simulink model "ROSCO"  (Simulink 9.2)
settings: Solver=VariableStepAuto  StartTime=0.0  StopTime=TMax  RelTol=1e-3
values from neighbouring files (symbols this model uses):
  OutList = [OutList    [runFAST.m]    (also in ROSCO2Matlab.m = [])
undefined symbols (not defined in the file or in its folder): cosd, DiscIntNeverNeededParam, F, Parameter, R, rpm2radps, simu, sind, strmatch
libraries: simulink x10
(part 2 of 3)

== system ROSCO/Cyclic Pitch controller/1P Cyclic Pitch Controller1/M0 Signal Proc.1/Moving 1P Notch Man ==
  Input : Inport
  GenSpeedIN : Inport  Port=2
  Gain : Gain  Gain=1/Parameter.Turbine.G * rpm2radps(1)
  Moving 1P Filt Manual : Subsystem
  Slow Low Pass for Param : DiscreteStateSpace  A=Parameter.Control.cIPC.dLPF_slow.a  B=Parameter.Control.cIPC.dLPF_slow.b  C=Parameter.Control.cIPC.dLPF_slow.c  D=Parameter.Control.cIPC.dLPF_slow.d  SampleTime=Parameter.Control.DT
  Output : Outport
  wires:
  GenSpeedIN/1 -> Slow Low Pass for Param/1
  Input/1 -> Moving 1P Filt Manual/1(u)
  Gain/1 -> Moving 1P Filt Manual/2(rot speed (rad/s))
  Slow Low Pass for Param/1 -> Gain/1
  Moving 1P Filt Manual/1(Out1) -> Output/1

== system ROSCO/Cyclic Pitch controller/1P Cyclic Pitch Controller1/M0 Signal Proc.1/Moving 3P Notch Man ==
  Input : Inport
  GenSpeedIN : Inport  Port=2
  Gain : Gain  Gain=1/Parameter.Turbine.G * rpm2radps(1) * 3
  Moving 3P Filt Manual : Subsystem
  Slow Low Pass for Param : DiscreteStateSpace  A=Parameter.Control.cIPC.dLPF_slow.a  B=Parameter.Control.cIPC.dLPF_slow.b  C=Parameter.Control.cIPC.dLPF_slow.c  D=Parameter.Control.cIPC.dLPF_slow.d  SampleTime=Parameter.Control.DT
  Output : Outport
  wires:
  Slow Low Pass for Param/1 -> Gain/1
  Gain/1 -> Moving 3P Filt Manual/2(rot speed (rad/s))
  Input/1 -> Moving 3P Filt Manual/1(u)
  GenSpeedIN/1 -> Slow Low Pass for Param/1
  Moving 3P Filt Manual/1(Out1) -> Output/1

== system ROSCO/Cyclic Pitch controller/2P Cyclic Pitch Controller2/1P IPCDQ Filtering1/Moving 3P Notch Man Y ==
  Input : Inport
  GenSpeedIN : Inport  Port=2
  Gain : Gain  Gain=1/Parameter.Turbine.G * rpm2radps(1) * 3
  Moving 3P Filt Manual : Subsystem
  Slow Low Pass for Param : DiscreteStateSpace  A=Parameter.Control.cIPC.dLPF_slow.a  B=Parameter.Control.cIPC.dLPF_slow.b  C=Parameter.Control.cIPC.dLPF_slow.c  D=Parameter.Control.cIPC.dLPF_slow.d  SampleTime=Parameter.Control.DT
  Output : Outport
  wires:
  Slow Low Pass for Param/1 -> Gain/1
  Gain/1 -> Moving 3P Filt Manual/2(rot speed (rad/s))
  Input/1 -> Moving 3P Filt Manual/1(u)
  GenSpeedIN/1 -> Slow Low Pass for Param/1
  Moving 3P Filt Manual/1(Out1) -> Output/1

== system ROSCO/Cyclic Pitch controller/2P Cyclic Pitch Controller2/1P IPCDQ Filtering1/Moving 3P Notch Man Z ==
  Input : Inport
  GenSpeedIN : Inport  Port=2
  Gain : Gain  Gain=1/Parameter.Turbine.G * rpm2radps(1) * 3
  Moving 3P Filt Manual : Subsystem
  Slow Low Pass for Param : DiscreteStateSpace  A=Parameter.Control.cIPC.dLPF_slow.a  B=Parameter.Control.cIPC.dLPF_slow.b  C=Parameter.Control.cIPC.dLPF_slow.c  D=Parameter.Control.cIPC.dLPF_slow.d  SampleTime=Parameter.Control.DT
  Output : Outport
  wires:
  Moving 3P Filt Manual/1(Out1) -> Output/1
  GenSpeedIN/1 -> Slow Low Pass for Param/1
  Input/1 -> Moving 3P Filt Manual/1(u)
  Gain/1 -> Moving 3P Filt Manual/2(rot speed (rad/s))
  Slow Low Pass for Param/1 -> Gain/1

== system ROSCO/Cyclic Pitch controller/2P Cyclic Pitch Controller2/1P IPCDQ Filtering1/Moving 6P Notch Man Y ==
  Input : Inport
  GenSpeedIN : Inport  Port=2
  Gain : Gain  Gain=1/Parameter.Turbine.G * rpm2radps(1) * 3
  Moving 6P Filt Manual : Subsystem
  Slow Low Pass for Param : DiscreteStateSpace  A=Parameter.Control.cIPC.dLPF_slow.a  B=Parameter.Control.cIPC.dLPF_slow.b  C=Parameter.Control.cIPC.dLPF_slow.c  D=Parameter.Control.cIPC.dLPF_slow.d  SampleTime=Parameter.Control.DT
  Output : Outport
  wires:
  Moving 6P Filt Manual/1(Out1) -> Output/1
  GenSpeedIN/1 -> Slow Low Pass for Param/1
  Input/1 -> Moving 6P Filt Manual/1(u)
  Gain/1 -> Moving 6P Filt Manual/2(rot speed (rad/s))
  Slow Low Pass for Param/1 -> Gain/1

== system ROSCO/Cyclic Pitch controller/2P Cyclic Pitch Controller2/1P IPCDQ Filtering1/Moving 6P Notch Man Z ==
  Input : Inport
  GenSpeedIN : Inport  Port=2
  Gain : Gain  Gain=1/Parameter.Turbine.G * rpm2radps(1) * 3
  Moving 6P Filt Manual : Subsystem
  Slow Low Pass for Param : DiscreteStateSpace  A=Parameter.Control.cIPC.dLPF_slow.a  B=Parameter.Control.cIPC.dLPF_slow.b  C=Parameter.Control.cIPC.dLPF_slow.c  D=Parameter.Control.cIPC.dLPF_slow.d  SampleTime=Parameter.Control.DT
  Output : Outport
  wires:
  Slow Low Pass for Param/1 -> Gain/1
  Gain/1 -> Moving 6P Filt Manual/2(rot speed (rad/s))
  Input/1 -> Moving 6P Filt Manual/1(u)
  GenSpeedIN/1 -> Slow Low Pass for Param/1
  Moving 6P Filt Manual/1(Out1) -> Output/1

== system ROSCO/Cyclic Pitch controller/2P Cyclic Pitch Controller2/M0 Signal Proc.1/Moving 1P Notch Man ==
  Input : Inport
  GenSpeedIN : Inport  Port=2
  Gain : Gain  Gain=1/Parameter.Turbine.G * rpm2radps(1)
  Moving 1P Filt Manual : Subsystem
  Slow Low Pass for Param : DiscreteStateSpace  A=Parameter.Control.cIPC.dLPF_slow.a  B=Parameter.Control.cIPC.dLPF_slow.b  C=Parameter.Control.cIPC.dLPF_slow.c  D=Parameter.Control.cIPC.dLPF_slow.d  SampleTime=Parameter.Control.DT
  Output : Outport
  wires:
  GenSpeedIN/1 -> Slow Low Pass for Param/1
  Input/1 -> Moving 1P Filt Manual/1(u)
  Gain/1 -> Moving 1P Filt Manual/2(rot speed (rad/s))
  Slow Low Pass for Param/1 -> Gain/1
  Moving 1P Filt Manual/1(Out1) -> Output/1

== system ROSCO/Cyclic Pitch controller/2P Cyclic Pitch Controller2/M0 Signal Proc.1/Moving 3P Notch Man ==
  Input : Inport
  GenSpeedIN : Inport  Port=2
  Gain : Gain  Gain=1/Parameter.Turbine.G * rpm2radps(1) * 3
  Moving 3P Filt Manual : Subsystem
  Slow Low Pass for Param : DiscreteStateSpace  A=Parameter.Control.cIPC.dLPF_slow.a  B=Parameter.Control.cIPC.dLPF_slow.b  C=Parameter.Control.cIPC.dLPF_slow.c  D=Parameter.Control.cIPC.dLPF_slow.d  SampleTime=Parameter.Control.DT
  Output : Outport
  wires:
  Slow Low Pass for Param/1 -> Gain/1
  Gain/1 -> Moving 3P Filt Manual/2(rot speed (rad/s))
  Input/1 -> Moving 3P Filt Manual/1(u)
  GenSpeedIN/1 -> Slow Low Pass for Param/1
  Moving 3P Filt Manual/1(Out1) -> Output/1

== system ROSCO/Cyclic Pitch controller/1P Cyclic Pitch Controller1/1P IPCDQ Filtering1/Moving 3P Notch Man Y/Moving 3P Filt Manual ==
  u : Inport
  rot speed (rad/s) : Inport  Port=2
  Den LPV : Subsystem
  Discrete Filter : DiscreteFilter  NumeratorSource=Input port  DenominatorSource=Input port  a0EqualsOne=on
  Num LPV : Subsystem
  Out1 : Outport
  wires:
  u/1 -> Discrete Filter/1
  Num LPV/1(b) -> Discrete Filter/2
  Discrete Filter/1 -> Out1/1
  rot speed (rad/s)/1 -> Den LPV/1(rot speed (rad/s)), Num LPV/1(rot speed (rad/s))
  Den LPV/1(a) -> Discrete Filter/3

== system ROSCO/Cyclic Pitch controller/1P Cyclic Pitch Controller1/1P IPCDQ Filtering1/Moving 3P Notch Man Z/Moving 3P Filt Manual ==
  u : Inport
  rot speed (rad/s) : Inport  Port=2
  Den LPV : Subsystem
  Discrete Filter : DiscreteFilter  NumeratorSource=Input port  DenominatorSource=Input port  a0EqualsOne=on
  Num LPV : Subsystem
  Out1 : Outport
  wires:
  Den LPV/1(a) -> Discrete Filter/3
  rot speed (rad/s)/1 -> Num LPV/1(rot speed (rad/s)), Den LPV/1(rot speed (rad/s))
  Discrete Filter/1 -> Out1/1
  Num LPV/1(b) -> Discrete Filter/2
  u/1 -> Discrete Filter/1

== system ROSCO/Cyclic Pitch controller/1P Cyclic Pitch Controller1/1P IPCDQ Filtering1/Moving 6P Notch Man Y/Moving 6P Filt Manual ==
  u : Inport
  rot speed (rad/s) : Inport  Port=2
  Den LPV : Subsystem
  Discrete Filter : DiscreteFilter  NumeratorSource=Input port  DenominatorSource=Input port  a0EqualsOne=on
  Num LPV : Subsystem
  Out1 : Outport
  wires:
  Den LPV/1(a) -> Discrete Filter/3
  rot speed (rad/s)/1 -> Num LPV/1(rot speed (rad/s)), Den LPV/1(rot speed (rad/s))
  Discrete Filter/1 -> Out1/1
  Num LPV/1(b) -> Discrete Filter/2
  u/1 -> Discrete Filter/1

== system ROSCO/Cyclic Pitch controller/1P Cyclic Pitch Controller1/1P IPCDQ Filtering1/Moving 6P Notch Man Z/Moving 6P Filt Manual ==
  u : Inport
  rot speed (rad/s) : Inport  Port=2
  Den LPV : Subsystem
  Discrete Filter : DiscreteFilter  NumeratorSource=Input port  DenominatorSource=Input port  a0EqualsOne=on
  Num LPV : Subsystem
  Out1 : Outport
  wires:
  u/1 -> Discrete Filter/1
  Num LPV/1(b) -> Discrete Filter/2
  Discrete Filter/1 -> Out1/1
  rot speed (rad/s)/1 -> Den LPV/1(rot speed (rad/s)), Num LPV/1(rot speed (rad/s))
  Den LPV/1(a) -> Discrete Filter/3

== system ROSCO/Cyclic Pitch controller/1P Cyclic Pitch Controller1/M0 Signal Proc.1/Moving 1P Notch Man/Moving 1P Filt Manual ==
  u : Inport
  rot speed (rad/s) : Inport  Port=2
  Den LPV : Subsystem
  Discrete Filter : DiscreteFilter  NumeratorSource=Input port  DenominatorSource=Input port  a0EqualsOne=on
  Num LPV : Subsystem
  Out1 : Outport
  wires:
  Den LPV/1(a) -> Discrete Filter/3
  rot speed (rad/s)/1 -> Num LPV/1(rot speed (rad/s)), Den LPV/1(rot speed (rad/s))
  Discrete Filter/1 -> Out1/1
  Num LPV/1(b) -> Discrete Filter/2
  u/1 -> Discrete Filter/1

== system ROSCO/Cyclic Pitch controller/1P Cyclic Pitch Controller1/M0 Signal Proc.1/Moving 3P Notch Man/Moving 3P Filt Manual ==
  u : Inport
  rot speed (rad/s) : Inport  Port=2
  Den LPV : Subsystem
  Discrete Filter : DiscreteFilter  NumeratorSource=Input port  DenominatorSource=Input port  a0EqualsOne=on
  Num LPV : Subsystem
  Out1 : Outport
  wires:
  u/1 -> Discrete Filter/1
  Num LPV/1(b) -> Discrete Filter/2
  Discrete Filter/1 -> Out1/1
  rot speed (rad/s)/1 -> Den LPV/1(rot speed (rad/s)), Num LPV/1(rot speed (rad/s))
  Den LPV/1(a) -> Discrete Filter/3

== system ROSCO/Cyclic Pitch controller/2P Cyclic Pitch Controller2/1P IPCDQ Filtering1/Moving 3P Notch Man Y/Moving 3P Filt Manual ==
  u : Inport
  rot speed (rad/s) : Inport  Port=2
  Den LPV : Subsystem
  Discrete Filter : DiscreteFilter  NumeratorSource=Input port  DenominatorSource=Input port  a0EqualsOne=on
  Num LPV : Subsystem
  Out1 : Outport
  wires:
  u/1 -> Discrete Filter/1
  Num LPV/1(b) -> Discrete Filter/2
  Discrete Filter/1 -> Out1/1
  rot speed (rad/s)/1 -> Den LPV/1(rot speed (rad/s)), Num LPV/1(rot speed (rad/s))
  Den LPV/1(a) -> Discrete Filter/3

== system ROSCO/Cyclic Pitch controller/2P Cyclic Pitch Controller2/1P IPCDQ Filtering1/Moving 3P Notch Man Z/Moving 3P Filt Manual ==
  u : Inport
  rot speed (rad/s) : Inport  Port=2
  Den LPV : Subsystem
  Discrete Filter : DiscreteFilter  NumeratorSource=Input port  DenominatorSource=Input port  a0EqualsOne=on
  Num LPV : Subsystem
  Out1 : Outport
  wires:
  Den LPV/1(a) -> Discrete Filter/3
  rot speed (rad/s)/1 -> Num LPV/1(rot speed (rad/s)), Den LPV/1(rot speed (rad/s))
  Discrete Filter/1 -> Out1/1
  Num LPV/1(b) -> Discrete Filter/2
  u/1 -> Discrete Filter/1

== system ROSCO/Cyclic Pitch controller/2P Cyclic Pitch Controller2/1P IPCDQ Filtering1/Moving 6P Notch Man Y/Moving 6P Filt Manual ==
  u : Inport
  rot speed (rad/s) : Inport  Port=2
  Den LPV : Subsystem
  Discrete Filter : DiscreteFilter  NumeratorSource=Input port  DenominatorSource=Input port  a0EqualsOne=on
  Num LPV : Subsystem
  Out1 : Outport
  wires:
  Den LPV/1(a) -> Discrete Filter/3
  rot speed (rad/s)/1 -> Num LPV/1(rot speed (rad/s)), Den LPV/1(rot speed (rad/s))
  Discrete Filter/1 -> Out1/1
  Num LPV/1(b) -> Discrete Filter/2
  u/1 -> Discrete Filter/1

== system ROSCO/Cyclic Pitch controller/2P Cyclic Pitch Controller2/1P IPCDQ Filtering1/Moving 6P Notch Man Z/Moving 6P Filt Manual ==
  u : Inport
  rot speed (rad/s) : Inport  Port=2
  Den LPV : Subsystem
  Discrete Filter : DiscreteFilter  NumeratorSource=Input port  DenominatorSource=Input port  a0EqualsOne=on
  Num LPV : Subsystem
  Out1 : Outport
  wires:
  u/1 -> Discrete Filter/1
  Num LPV/1(b) -> Discrete Filter/2
  Discrete Filter/1 -> Out1/1
  rot speed (rad/s)/1 -> Den LPV/1(rot speed (rad/s)), Num LPV/1(rot speed (rad/s))
  Den LPV/1(a) -> Discrete Filter/3

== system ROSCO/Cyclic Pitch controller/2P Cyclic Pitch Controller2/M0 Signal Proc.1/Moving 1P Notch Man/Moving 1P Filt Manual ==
  u : Inport
  rot speed (rad/s) : Inport  Port=2
  Den LPV : Subsystem
  Discrete Filter : DiscreteFilter  NumeratorSource=Input port  DenominatorSource=Input port  a0EqualsOne=on
  Num LPV : Subsystem
  Out1 : Outport
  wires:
  Den LPV/1(a) -> Discrete Filter/3
  rot speed (rad/s)/1 -> Num LPV/1(rot speed (rad/s)), Den LPV/1(rot speed (rad/s))
  Discrete Filter/1 -> Out1/1
  Num LPV/1(b) -> Discrete Filter/2
  u/1 -> Discrete Filter/1

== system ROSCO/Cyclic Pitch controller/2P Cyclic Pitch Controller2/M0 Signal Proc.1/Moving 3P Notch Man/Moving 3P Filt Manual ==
  u : Inport
  rot speed (rad/s) : Inport  Port=2
  Den LPV : Subsystem
  Discrete Filter : DiscreteFilter  NumeratorSource=Input port  DenominatorSource=Input port  a0EqualsOne=on
  Num LPV : Subsystem
  Out1 : Outport
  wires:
  u/1 -> Discrete Filter/1
  Num LPV/1(b) -> Discrete Filter/2
  Discrete Filter/1 -> Out1/1
  rot speed (rad/s)/1 -> Den LPV/1(rot speed (rad/s)), Num LPV/1(rot speed (rad/s))
  Den LPV/1(a) -> Discrete Filter/3

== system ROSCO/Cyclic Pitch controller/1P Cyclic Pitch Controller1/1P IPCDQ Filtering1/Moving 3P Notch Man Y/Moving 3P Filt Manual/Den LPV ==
  rot speed (rad/s) : Inport
  1-D Lookup Table : Lookup_n-D  NumberOfTableDimensions=1  BreakpointsForDimension1=Parameter.Control.cIPC.PSM0_NF_3P.om_3P  BeginIndexSearchUsingPreviousIndexResult=on  Table=Parameter.Control.cIPC.PSM0_NF_3P.a_2  ExtrapMethod=Clip  InternalRulePriority=Speed  RndMeth=Simplest
  1-D Lookup Table1 : Lookup_n-D  NumberOfTableDimensions=1  BreakpointsForDimension1=Parameter.Control.cIPC.PSM0_NF_3P.om_3P  BeginIndexSearchUsingPreviousIndexResult=on  Table=Parameter.Control.cIPC.PSM0_NF_3P.a_1  ExtrapMethod=Clip  InternalRulePriority=Speed  RndMeth=Simplest
  1-D Lookup Table2 : Lookup_n-D  NumberOfTableDimensions=1  BreakpointsForDimension1=Parameter.Control.cIPC.PSM0_NF_3P.om_3P  BeginIndexSearchUsingPreviousIndexResult=on  Table=Parameter.Control.cIPC.PSM0_NF_3P.a_0  ExtrapMethod=Clip  InternalRulePriority=Speed  RndMeth=Simplest
  Mux : Mux  Inputs=3
  a : Outport
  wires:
  1-D Lookup Table/1 -> Mux/1
  1-D Lookup Table1/1 -> Mux/2
  Mux/1 -> a/1
  rot speed (rad/s)/1 -> 1-D Lookup Table2/1, 1-D Lookup Table/1, 1-D Lookup Table1/1
  1-D Lookup Table2/1 -> Mux/3

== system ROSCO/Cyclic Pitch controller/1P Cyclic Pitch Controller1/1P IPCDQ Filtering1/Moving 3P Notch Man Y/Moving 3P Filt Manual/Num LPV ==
  rot speed (rad/s) : Inport
  1-D Lookup Table : Lookup_n-D  NumberOfTableDimensions=1  BreakpointsForDimension1=Parameter.Control.cIPC.PSM0_NF_3P.om_3P  BeginIndexSearchUsingPreviousIndexResult=on  Table=Parameter.Control.cIPC.PSM0_NF_3P.b_2  ExtrapMethod=Clip  InternalRulePriority=Speed  RndMeth=Simplest
  1-D Lookup Table1 : Lookup_n-D  NumberOfTableDimensions=1  BreakpointsForDimension1=Parameter.Control.cIPC.PSM0_NF_3P.om_3P  BeginIndexSearchUsingPreviousIndexResult=on  Table=Parameter.Control.cIPC.PSM0_NF_3P.b_1  ExtrapMethod=Clip  InternalRulePriority=Speed  RndMeth=Simplest
  1-D Lookup Table2 : Lookup_n-D  NumberOfTableDimensions=1  BreakpointsForDimension1=Parameter.Control.cIPC.PSM0_NF_3P.om_3P  BeginIndexSearchUsingPreviousIndexResult=on  Table=Parameter.Control.cIPC.PSM0_NF_3P.b_0  ExtrapMethod=Clip  InternalRulePriority=Speed  RndMeth=Simplest
  Mux : Mux  Inputs=3
  b : Outport
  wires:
  1-D Lookup Table2/1 -> Mux/3
  rot speed (rad/s)/1 -> 1-D Lookup Table1/1, 1-D Lookup Table/1, 1-D Lookup Table2/1
  Mux/1 -> b/1
  1-D Lookup Table1/1 -> Mux/2
  1-D Lookup Table/1 -> Mux/1

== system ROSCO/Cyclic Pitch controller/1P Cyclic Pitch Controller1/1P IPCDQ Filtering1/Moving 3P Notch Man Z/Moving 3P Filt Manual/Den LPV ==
  rot speed (rad/s) : Inport
  1-D Lookup Table : Lookup_n-D  NumberOfTableDimensions=1  BreakpointsForDimension1=Parameter.Control.cIPC.PSM0_NF_3P.om_3P  BeginIndexSearchUsingPreviousIndexResult=on  Table=Parameter.Control.cIPC.PSM0_NF_3P.a_2  ExtrapMethod=Clip  InternalRulePriority=Speed  RndMeth=Simplest
  1-D Lookup Table1 : Lookup_n-D  NumberOfTableDimensions=1  BreakpointsForDimension1=Parameter.Control.cIPC.PSM0_NF_3P.om_3P  BeginIndexSearchUsingPreviousIndexResult=on  Table=Parameter.Control.cIPC.PSM0_NF_3P.a_1  ExtrapMethod=Clip  InternalRulePriority=Speed  RndMeth=Simplest
  1-D Lookup Table2 : Lookup_n-D  NumberOfTableDimensions=1  BreakpointsForDimension1=Parameter.Control.cIPC.PSM0_NF_3P.om_3P  BeginIndexSearchUsingPreviousIndexResult=on  Table=Parameter.Control.cIPC.PSM0_NF_3P.a_0  ExtrapMethod=Clip  InternalRulePriority=Speed  RndMeth=Simplest
  Mux : Mux  Inputs=3
  a : Outport
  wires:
  1-D Lookup Table2/1 -> Mux/3
  rot speed (rad/s)/1 -> 1-D Lookup Table1/1, 1-D Lookup Table/1, 1-D Lookup Table2/1
  Mux/1 -> a/1
  1-D Lookup Table1/1 -> Mux/2
  1-D Lookup Table/1 -> Mux/1

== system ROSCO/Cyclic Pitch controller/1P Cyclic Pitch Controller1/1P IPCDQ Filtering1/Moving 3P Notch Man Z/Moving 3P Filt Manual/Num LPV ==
  rot speed (rad/s) : Inport
  1-D Lookup Table : Lookup_n-D  NumberOfTableDimensions=1  BreakpointsForDimension1=Parameter.Control.cIPC.PSM0_NF_3P.om_3P  BeginIndexSearchUsingPreviousIndexResult=on  Table=Parameter.Control.cIPC.PSM0_NF_3P.b_2  ExtrapMethod=Clip  InternalRulePriority=Speed  RndMeth=Simplest
  1-D Lookup Table1 : Lookup_n-D  NumberOfTableDimensions=1  BreakpointsForDimension1=Parameter.Control.cIPC.PSM0_NF_3P.om_3P  BeginIndexSearchUsingPreviousIndexResult=on  Table=Parameter.Control.cIPC.PSM0_NF_3P.b_1  ExtrapMethod=Clip  InternalRulePriority=Speed  RndMeth=Simplest
  1-D Lookup Table2 : Lookup_n-D  NumberOfTableDimensions=1  BreakpointsForDimension1=Parameter.Control.cIPC.PSM0_NF_3P.om_3P  BeginIndexSearchUsingPreviousIndexResult=on  Table=Parameter.Control.cIPC.PSM0_NF_3P.b_0  ExtrapMethod=Clip  InternalRulePriority=Speed  RndMeth=Simplest
  Mux : Mux  Inputs=3
  b : Outport
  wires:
  1-D Lookup Table/1 -> Mux/1
  1-D Lookup Table1/1 -> Mux/2
  Mux/1 -> b/1
  rot speed (rad/s)/1 -> 1-D Lookup Table2/1, 1-D Lookup Table/1, 1-D Lookup Table1/1
  1-D Lookup Table2/1 -> Mux/3

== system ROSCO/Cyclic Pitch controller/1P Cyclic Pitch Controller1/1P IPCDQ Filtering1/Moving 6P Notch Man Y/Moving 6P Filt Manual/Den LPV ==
  rot speed (rad/s) : Inport
  1-D Lookup Table : Lookup_n-D  NumberOfTableDimensions=1  BreakpointsForDimension1=Parameter.Control.cIPC.PSM0_NF_6P.om_6P  BeginIndexSearchUsingPreviousIndexResult=on  Table=Parameter.Control.cIPC.PSM0_NF_6P.a_2  ExtrapMethod=Clip  InternalRulePriority=Speed  RndMeth=Simplest
  1-D Lookup Table1 : Lookup_n-D  NumberOfTableDimensions=1  BreakpointsForDimension1=Parameter.Control.cIPC.PSM0_NF_6P.om_6P  BeginIndexSearchUsingPreviousIndexResult=on  Table=Parameter.Control.cIPC.PSM0_NF_6P.a_1  ExtrapMethod=Clip  InternalRulePriority=Speed  RndMeth=Simplest
  1-D Lookup Table2 : Lookup_n-D  NumberOfTableDimensions=1  BreakpointsForDimension1=Parameter.Control.cIPC.PSM0_NF_6P.om_6P  BeginIndexSearchUsingPreviousIndexResult=on  Table=Parameter.Control.cIPC.PSM0_NF_6P.a_0  ExtrapMethod=Clip  InternalRulePriority=Speed  RndMeth=Simplest
  Mux : Mux  Inputs=3
  a : Outport
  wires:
  1-D Lookup Table2/1 -> Mux/3
  rot speed (rad/s)/1 -> 1-D Lookup Table1/1, 1-D Lookup Table/1, 1-D Lookup Table2/1
  Mux/1 -> a/1
  1-D Lookup Table1/1 -> Mux/2
  1-D Lookup Table/1 -> Mux/1

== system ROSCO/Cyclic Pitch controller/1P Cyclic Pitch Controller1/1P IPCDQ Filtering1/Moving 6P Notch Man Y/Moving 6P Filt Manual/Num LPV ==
  rot speed (rad/s) : Inport
  1-D Lookup Table : Lookup_n-D  NumberOfTableDimensions=1  BreakpointsForDimension1=Parameter.Control.cIPC.PSM0_NF_6P.om_6P  BeginIndexSearchUsingPreviousIndexResult=on  Table=Parameter.Control.cIPC.PSM0_NF_6P.b_2  ExtrapMethod=Clip  InternalRulePriority=Speed  RndMeth=Simplest
  1-D Lookup Table1 : Lookup_n-D  NumberOfTableDimensions=1  BreakpointsForDimension1=Parameter.Control.cIPC.PSM0_NF_6P.om_6P  BeginIndexSearchUsingPreviousIndexResult=on  Table=Parameter.Control.cIPC.PSM0_NF_6P.b_1  ExtrapMethod=Clip  InternalRulePriority=Speed  RndMeth=Simplest
  1-D Lookup Table2 : Lookup_n-D  NumberOfTableDimensions=1  BreakpointsForDimension1=Parameter.Control.cIPC.PSM0_NF_6P.om_6P  BeginIndexSearchUsingPreviousIndexResult=on  Table=Parameter.Control.cIPC.PSM0_NF_6P.b_0  ExtrapMethod=Clip  InternalRulePriority=Speed  RndMeth=Simplest
  Mux : Mux  Inputs=3
  b : Outport
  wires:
  1-D Lookup Table/1 -> Mux/1
  1-D Lookup Table1/1 -> Mux/2
  Mux/1 -> b/1
  rot speed (rad/s)/1 -> 1-D Lookup Table2/1, 1-D Lookup Table1/1, 1-D Lookup Table/1
  1-D Lookup Table2/1 -> Mux/3

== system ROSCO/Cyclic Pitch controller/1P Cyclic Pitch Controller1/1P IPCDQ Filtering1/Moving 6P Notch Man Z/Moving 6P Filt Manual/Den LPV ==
  rot speed (rad/s) : Inport
  1-D Lookup Table : Lookup_n-D  NumberOfTableDimensions=1  BreakpointsForDimension1=Parameter.Control.cIPC.PSM0_NF_6P.om_6P  BeginIndexSearchUsingPreviousIndexResult=on  Table=Parameter.Control.cIPC.PSM0_NF_6P.a_2  ExtrapMethod=Clip  InternalRulePriority=Speed  RndMeth=Simplest
  1-D Lookup Table1 : Lookup_n-D  NumberOfTableDimensions=1  BreakpointsForDimension1=Parameter.Control.cIPC.PSM0_NF_6P.om_6P  BeginIndexSearchUsingPreviousIndexResult=on  Table=Parameter.Control.cIPC.PSM0_NF_6P.a_1  ExtrapMethod=Clip  InternalRulePriority=Speed  RndMeth=Simplest
  1-D Lookup Table2 : Lookup_n-D  NumberOfTableDimensions=1  BreakpointsForDimension1=Parameter.Control.cIPC.PSM0_NF_6P.om_6P  BeginIndexSearchUsingPreviousIndexResult=on  Table=Parameter.Control.cIPC.PSM0_NF_6P.a_0  ExtrapMethod=Clip  InternalRulePriority=Speed  RndMeth=Simplest
  Mux : Mux  Inputs=3
  a : Outport
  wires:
  1-D Lookup Table/1 -> Mux/1
  1-D Lookup Table1/1 -> Mux/2
  Mux/1 -> a/1
  rot speed (rad/s)/1 -> 1-D Lookup Table2/1, 1-D Lookup Table/1, 1-D Lookup Table1/1
  1-D Lookup Table2/1 -> Mux/3

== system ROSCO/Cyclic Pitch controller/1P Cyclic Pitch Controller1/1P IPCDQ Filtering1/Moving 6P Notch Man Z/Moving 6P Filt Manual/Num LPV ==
  rot speed (rad/s) : Inport
  1-D Lookup Table : Lookup_n-D  NumberOfTableDimensions=1  BreakpointsForDimension1=Parameter.Control.cIPC.PSM0_NF_6P.om_6P  BeginIndexSearchUsingPreviousIndexResult=on  Table=Parameter.Control.cIPC.PSM0_NF_6P.b_2  ExtrapMethod=Clip  InternalRulePriority=Speed  RndMeth=Simplest
  1-D Lookup Table1 : Lookup_n-D  NumberOfTableDimensions=1  BreakpointsForDimension1=Parameter.Control.cIPC.PSM0_NF_6P.om_6P  BeginIndexSearchUsingPreviousIndexResult=on  Table=Parameter.Control.cIPC.PSM0_NF_6P.b_1  ExtrapMethod=Clip  InternalRulePriority=Speed  RndMeth=Simplest
  1-D Lookup Table2 : Lookup_n-D  NumberOfTableDimensions=1  BreakpointsForDimension1=Parameter.Control.cIPC.PSM0_NF_6P.om_6P  BeginIndexSearchUsingPreviousIndexResult=on  Table=Parameter.Control.cIPC.PSM0_NF_6P.b_0  ExtrapMethod=Clip  InternalRulePriority=Speed  RndMeth=Simplest
  Mux : Mux  Inputs=3
  b : Outport
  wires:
  1-D Lookup Table2/1 -> Mux/3
  rot speed (rad/s)/1 -> 1-D Lookup Table1/1, 1-D Lookup Table/1, 1-D Lookup Table2/1
  Mux/1 -> b/1
  1-D Lookup Table1/1 -> Mux/2
  1-D Lookup Table/1 -> Mux/1

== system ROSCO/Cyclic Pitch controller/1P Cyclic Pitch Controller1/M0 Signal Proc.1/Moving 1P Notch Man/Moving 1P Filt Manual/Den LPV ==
  rot speed (rad/s) : Inport
  1-D Lookup Table : Lookup_n-D  NumberOfTableDimensions=1  BreakpointsForDimension1=Parameter.Control.cIPC.PSM0_NF_1P.om_1P  BeginIndexSearchUsingPreviousIndexResult=on  Table=Parameter.Control.cIPC.PSM0_NF_1P.a_2  ExtrapMethod=Clip  InternalRulePriority=Speed  RndMeth=Simplest
  1-D Lookup Table1 : Lookup_n-D  NumberOfTableDimensions=1  BreakpointsForDimension1=Parameter.Control.cIPC.PSM0_NF_1P.om_1P  BeginIndexSearchUsingPreviousIndexResult=on  Table=Parameter.Control.cIPC.PSM0_NF_1P.a_1  ExtrapMethod=Clip  InternalRulePriority=Speed  RndMeth=Simplest
  1-D Lookup Table2 : Lookup_n-D  NumberOfTableDimensions=1  BreakpointsForDimension1=Parameter.Control.cIPC.PSM0_NF_1P.om_1P  BeginIndexSearchUsingPreviousIndexResult=on  Table=Parameter.Control.cIPC.PSM0_NF_1P.a_0  ExtrapMethod=Clip  InternalRulePriority=Speed  RndMeth=Simplest
  Mux : Mux  Inputs=3
  a : Outport
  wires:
  1-D Lookup Table2/1 -> Mux/3
  rot speed (rad/s)/1 -> 1-D Lookup Table1/1, 1-D Lookup Table/1, 1-D Lookup Table2/1
  Mux/1 -> a/1
  1-D Lookup Table1/1 -> Mux/2
  1-D Lookup Table/1 -> Mux/1

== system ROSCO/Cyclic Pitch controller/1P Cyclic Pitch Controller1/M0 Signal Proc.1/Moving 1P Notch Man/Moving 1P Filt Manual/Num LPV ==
  rot speed (rad/s) : Inport
  1-D Lookup Table : Lookup_n-D  NumberOfTableDimensions=1  BreakpointsForDimension1=Parameter.Control.cIPC.PSM0_NF_1P.om_1P  BeginIndexSearchUsingPreviousIndexResult=on  Table=Parameter.Control.cIPC.PSM0_NF_1P.b_2  ExtrapMethod=Clip  InternalRulePriority=Speed  RndMeth=Simplest
  1-D Lookup Table1 : Lookup_n-D  NumberOfTableDimensions=1  BreakpointsForDimension1=Parameter.Control.cIPC.PSM0_NF_1P.om_1P  BeginIndexSearchUsingPreviousIndexResult=on  Table=Parameter.Control.cIPC.PSM0_NF_1P.b_1  ExtrapMethod=Clip  InternalRulePriority=Speed  RndMeth=Simplest
  1-D Lookup Table2 : Lookup_n-D  NumberOfTableDimensions=1  BreakpointsForDimension1=Parameter.Control.cIPC.PSM0_NF_1P.om_1P  BeginIndexSearchUsingPreviousIndexResult=on  Table=Parameter.Control.cIPC.PSM0_NF_1P.b_0  ExtrapMethod=Clip  InternalRulePriority=Speed  RndMeth=Simplest
  Mux : Mux  Inputs=3
  b : Outport
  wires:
  1-D Lookup Table/1 -> Mux/1
  1-D Lookup Table1/1 -> Mux/2
  Mux/1 -> b/1
  rot speed (rad/s)/1 -> 1-D Lookup Table2/1, 1-D Lookup Table/1, 1-D Lookup Table1/1
  1-D Lookup Table2/1 -> Mux/3

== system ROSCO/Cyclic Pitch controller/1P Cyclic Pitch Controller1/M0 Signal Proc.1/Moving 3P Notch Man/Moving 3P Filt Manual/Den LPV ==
  rot speed (rad/s) : Inport
  1-D Lookup Table : Lookup_n-D  NumberOfTableDimensions=1  BreakpointsForDimension1=Parameter.Control.cIPC.PSM0_NF_3P.om_3P  BeginIndexSearchUsingPreviousIndexResult=on  Table=Parameter.Control.cIPC.PSM0_NF_3P.a_2  ExtrapMethod=Clip  InternalRulePriority=Speed  RndMeth=Simplest
  1-D Lookup Table1 : Lookup_n-D  NumberOfTableDimensions=1  BreakpointsForDimension1=Parameter.Control.cIPC.PSM0_NF_3P.om_3P  BeginIndexSearchUsingPreviousIndexResult=on  Table=Parameter.Control.cIPC.PSM0_NF_3P.a_1  ExtrapMethod=Clip  InternalRulePriority=Speed  RndMeth=Simplest
  1-D Lookup Table2 : Lookup_n-D  NumberOfTableDimensions=1  BreakpointsForDimension1=Parameter.Control.cIPC.PSM0_NF_3P.om_3P  BeginIndexSearchUsingPreviousIndexResult=on  Table=Parameter.Control.cIPC.PSM0_NF_3P.a_0  ExtrapMethod=Clip  InternalRulePriority=Speed  RndMeth=Simplest
  Mux : Mux  Inputs=3
  a : Outport
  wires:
  1-D Lookup Table/1 -> Mux/1
  1-D Lookup Table1/1 -> Mux/2
  Mux/1 -> a/1
  rot speed (rad/s)/1 -> 1-D Lookup Table2/1, 1-D Lookup Table/1, 1-D Lookup Table1/1
  1-D Lookup Table2/1 -> Mux/3

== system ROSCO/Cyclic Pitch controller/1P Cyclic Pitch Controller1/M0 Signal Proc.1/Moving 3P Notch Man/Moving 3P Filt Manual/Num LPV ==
  rot speed (rad/s) : Inport
  1-D Lookup Table : Lookup_n-D  NumberOfTableDimensions=1  BreakpointsForDimension1=Parameter.Control.cIPC.PSM0_NF_3P.om_3P  BeginIndexSearchUsingPreviousIndexResult=on  Table=Parameter.Control.cIPC.PSM0_NF_3P.b_2  ExtrapMethod=Clip  InternalRulePriority=Speed  RndMeth=Simplest
  1-D Lookup Table1 : Lookup_n-D  NumberOfTableDimensions=1  BreakpointsForDimension1=Parameter.Control.cIPC.PSM0_NF_3P.om_3P  BeginIndexSearchUsingPreviousIndexResult=on  Table=Parameter.Control.cIPC.PSM0_NF_3P.b_1  ExtrapMethod=Clip  InternalRulePriority=Speed  RndMeth=Simplest
  1-D Lookup Table2 : Lookup_n-D  NumberOfTableDimensions=1  BreakpointsForDimension1=Parameter.Control.cIPC.PSM0_NF_3P.om_3P  BeginIndexSearchUsingPreviousIndexResult=on  Table=Parameter.Control.cIPC.PSM0_NF_3P.b_0  ExtrapMethod=Clip  InternalRulePriority=Speed  RndMeth=Simplest
  Mux : Mux  Inputs=3
  b : Outport
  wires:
  1-D Lookup Table2/1 -> Mux/3
  rot speed (rad/s)/1 -> 1-D Lookup Table1/1, 1-D Lookup Table/1, 1-D Lookup Table2/1
  Mux/1 -> b/1
  1-D Lookup Table1/1 -> Mux/2
  1-D Lookup Table/1 -> Mux/1

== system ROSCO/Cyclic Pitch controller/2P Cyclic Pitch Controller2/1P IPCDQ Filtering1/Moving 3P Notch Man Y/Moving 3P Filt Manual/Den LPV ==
  rot speed (rad/s) : Inport
  1-D Lookup Table : Lookup_n-D  NumberOfTableDimensions=1  BreakpointsForDimension1=Parameter.Control.cIPC.PSM0_NF_3P.om_3P  BeginIndexSearchUsingPreviousIndexResult=on  Table=Parameter.Control.cIPC.PSM0_NF_3P.a_2  ExtrapMethod=Clip  InternalRulePriority=Speed  RndMeth=Simplest
  1-D Lookup Table1 : Lookup_n-D  NumberOfTableDimensions=1  BreakpointsForDimension1=Parameter.Control.cIPC.PSM0_NF_3P.om_3P  BeginIndexSearchUsingPreviousIndexResult=on  Table=Parameter.Control.cIPC.PSM0_NF_3P.a_1  ExtrapMethod=Clip  InternalRulePriority=Speed  RndMeth=Simplest
  1-D Lookup Table2 : Lookup_n-D  NumberOfTableDimensions=1  BreakpointsForDimension1=Parameter.Control.cIPC.PSM0_NF_3P.om_3P  BeginIndexSearchUsingPreviousIndexResult=on  Table=Parameter.Control.cIPC.PSM0_NF_3P.a_0  ExtrapMethod=Clip  InternalRulePriority=Speed  RndMeth=Simplest
  Mux : Mux  Inputs=3
  a : Outport
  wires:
  1-D Lookup Table/1 -> Mux/1
  1-D Lookup Table1/1 -> Mux/2
  Mux/1 -> a/1
  rot speed (rad/s)/1 -> 1-D Lookup Table2/1, 1-D Lookup Table/1, 1-D Lookup Table1/1
  1-D Lookup Table2/1 -> Mux/3

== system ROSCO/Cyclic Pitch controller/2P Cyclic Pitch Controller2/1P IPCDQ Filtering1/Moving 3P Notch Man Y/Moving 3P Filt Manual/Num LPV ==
  rot speed (rad/s) : Inport
  1-D Lookup Table : Lookup_n-D  NumberOfTableDimensions=1  BreakpointsForDimension1=Parameter.Control.cIPC.PSM0_NF_3P.om_3P  BeginIndexSearchUsingPreviousIndexResult=on  Table=Parameter.Control.cIPC.PSM0_NF_3P.b_2  ExtrapMethod=Clip  InternalRulePriority=Speed  RndMeth=Simplest
  1-D Lookup Table1 : Lookup_n-D  NumberOfTableDimensions=1  BreakpointsForDimension1=Parameter.Control.cIPC.PSM0_NF_3P.om_3P  BeginIndexSearchUsingPreviousIndexResult=on  Table=Parameter.Control.cIPC.PSM0_NF_3P.b_1  ExtrapMethod=Clip  InternalRulePriority=Speed  RndMeth=Simplest
  1-D Lookup Table2 : Lookup_n-D  NumberOfTableDimensions=1  BreakpointsForDimension1=Parameter.Control.cIPC.PSM0_NF_3P.om_3P  BeginIndexSearchUsingPreviousIndexResult=on  Table=Parameter.Control.cIPC.PSM0_NF_3P.b_0  ExtrapMethod=Clip  InternalRulePriority=Speed  RndMeth=Simplest
  Mux : Mux  Inputs=3
  b : Outport
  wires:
  1-D Lookup Table2/1 -> Mux/3
  rot speed (rad/s)/1 -> 1-D Lookup Table1/1, 1-D Lookup Table/1, 1-D Lookup Table2/1
  Mux/1 -> b/1
  1-D Lookup Table1/1 -> Mux/2
  1-D Lookup Table/1 -> Mux/1

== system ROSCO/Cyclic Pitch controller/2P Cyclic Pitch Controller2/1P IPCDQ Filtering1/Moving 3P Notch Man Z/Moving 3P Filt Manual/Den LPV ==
  rot speed (rad/s) : Inport
  1-D Lookup Table : Lookup_n-D  NumberOfTableDimensions=1  BreakpointsForDimension1=Parameter.Control.cIPC.PSM0_NF_3P.om_3P  BeginIndexSearchUsingPreviousIndexResult=on  Table=Parameter.Control.cIPC.PSM0_NF_3P.a_2  ExtrapMethod=Clip  InternalRulePriority=Speed  RndMeth=Simplest
  1-D Lookup Table1 : Lookup_n-D  NumberOfTableDimensions=1  BreakpointsForDimension1=Parameter.Control.cIPC.PSM0_NF_3P.om_3P  BeginIndexSearchUsingPreviousIndexResult=on  Table=Parameter.Control.cIPC.PSM0_NF_3P.a_1  ExtrapMethod=Clip  InternalRulePriority=Speed  RndMeth=Simplest
  1-D Lookup Table2 : Lookup_n-D  NumberOfTableDimensions=1  BreakpointsForDimension1=Parameter.Control.cIPC.PSM0_NF_3P.om_3P  BeginIndexSearchUsingPreviousIndexResult=on  Table=Parameter.Control.cIPC.PSM0_NF_3P.a_0  ExtrapMethod=Clip  InternalRulePriority=Speed  RndMeth=Simplest
  Mux : Mux  Inputs=3
  a : Outport
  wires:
  1-D Lookup Table2/1 -> Mux/3
  rot speed (rad/s)/1 -> 1-D Lookup Table1/1, 1-D Lookup Table/1, 1-D Lookup Table2/1
  Mux/1 -> a/1
  1-D Lookup Table1/1 -> Mux/2
  1-D Lookup Table/1 -> Mux/1

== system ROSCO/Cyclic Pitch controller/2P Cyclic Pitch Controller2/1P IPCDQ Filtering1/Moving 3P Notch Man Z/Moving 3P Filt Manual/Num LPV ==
  rot speed (rad/s) : Inport
  1-D Lookup Table : Lookup_n-D  NumberOfTableDimensions=1  BreakpointsForDimension1=Parameter.Control.cIPC.PSM0_NF_3P.om_3P  BeginIndexSearchUsingPreviousIndexResult=on  Table=Parameter.Control.cIPC.PSM0_NF_3P.b_2  ExtrapMethod=Clip  InternalRulePriority=Speed  RndMeth=Simplest
  1-D Lookup Table1 : Lookup_n-D  NumberOfTableDimensions=1  BreakpointsForDimension1=Parameter.Control.cIPC.PSM0_NF_3P.om_3P  BeginIndexSearchUsingPreviousIndexResult=on  Table=Parameter.Control.cIPC.PSM0_NF_3P.b_1  ExtrapMethod=Clip  InternalRulePriority=Speed  RndMeth=Simplest
  1-D Lookup Table2 : Lookup_n-D  NumberOfTableDimensions=1  BreakpointsForDimension1=Parameter.Control.cIPC.PSM0_NF_3P.om_3P  BeginIndexSearchUsingPreviousIndexResult=on  Table=Parameter.Control.cIPC.PSM0_NF_3P.b_0  ExtrapMethod=Clip  InternalRulePriority=Speed  RndMeth=Simplest
  Mux : Mux  Inputs=3
  b : Outport
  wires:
  1-D Lookup Table/1 -> Mux/1
  1-D Lookup Table1/1 -> Mux/2
  Mux/1 -> b/1
  rot speed (rad/s)/1 -> 1-D Lookup Table2/1, 1-D Lookup Table/1, 1-D Lookup Table1/1
  1-D Lookup Table2/1 -> Mux/3

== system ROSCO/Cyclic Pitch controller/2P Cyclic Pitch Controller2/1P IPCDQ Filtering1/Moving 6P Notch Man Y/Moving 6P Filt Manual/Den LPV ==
  rot speed (rad/s) : Inport
  1-D Lookup Table : Lookup_n-D  NumberOfTableDimensions=1  BreakpointsForDimension1=Parameter.Control.cIPC.PSM0_NF_6P.om_6P  BeginIndexSearchUsingPreviousIndexResult=on  Table=Parameter.Control.cIPC.PSM0_NF_6P.a_2  ExtrapMethod=Clip  InternalRulePriority=Speed  RndMeth=Simplest
  1-D Lookup Table1 : Lookup_n-D  NumberOfTableDimensions=1  BreakpointsForDimension1=Parameter.Control.cIPC.PSM0_NF_6P.om_6P  BeginIndexSearchUsingPreviousIndexResult=on  Table=Parameter.Control.cIPC.PSM0_NF_6P.a_1  ExtrapMethod=Clip  InternalRulePriority=Speed  RndMeth=Simplest
  1-D Lookup Table2 : Lookup_n-D  NumberOfTableDimensions=1  BreakpointsForDimension1=Parameter.Control.cIPC.PSM0_NF_6P.om_6P  BeginIndexSearchUsingPreviousIndexResult=on  Table=Parameter.Control.cIPC.PSM0_NF_6P.a_0  ExtrapMethod=Clip  InternalRulePriority=Speed  RndMeth=Simplest
  Mux : Mux  Inputs=3
  a : Outport
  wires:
  1-D Lookup Table2/1 -> Mux/3
  rot speed (rad/s)/1 -> 1-D Lookup Table1/1, 1-D Lookup Table/1, 1-D Lookup Table2/1
  Mux/1 -> a/1
  1-D Lookup Table1/1 -> Mux/2
  1-D Lookup Table/1 -> Mux/1

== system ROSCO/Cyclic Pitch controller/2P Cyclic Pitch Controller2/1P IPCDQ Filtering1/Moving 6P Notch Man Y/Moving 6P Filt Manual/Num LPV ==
  rot speed (rad/s) : Inport
  1-D Lookup Table : Lookup_n-D  NumberOfTableDimensions=1  BreakpointsForDimension1=Parameter.Control.cIPC.PSM0_NF_6P.om_6P  BeginIndexSearchUsingPreviousIndexResult=on  Table=Parameter.Control.cIPC.PSM0_NF_6P.b_2  ExtrapMethod=Clip  InternalRulePriority=Speed  RndMeth=Simplest
  1-D Lookup Table1 : Lookup_n-D  NumberOfTableDimensions=1  BreakpointsForDimension1=Parameter.Control.cIPC.PSM0_NF_6P.om_6P  BeginIndexSearchUsingPreviousIndexResult=on  Table=Parameter.Control.cIPC.PSM0_NF_6P.b_1  ExtrapMethod=Clip  InternalRulePriority=Speed  RndMeth=Simplest
  1-D Lookup Table2 : Lookup_n-D  NumberOfTableDimensions=1  BreakpointsForDimension1=Parameter.Control.cIPC.PSM0_NF_6P.om_6P  BeginIndexSearchUsingPreviousIndexResult=on  Table=Parameter.Control.cIPC.PSM0_NF_6P.b_0  ExtrapMethod=Clip  InternalRulePriority=Speed  RndMeth=Simplest
  Mux : Mux  Inputs=3
  b : Outport
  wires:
  1-D Lookup Table/1 -> Mux/1
  1-D Lookup Table1/1 -> Mux/2
  Mux/1 -> b/1
  rot speed (rad/s)/1 -> 1-D Lookup Table2/1, 1-D Lookup Table1/1, 1-D Lookup Table/1
  1-D Lookup Table2/1 -> Mux/3

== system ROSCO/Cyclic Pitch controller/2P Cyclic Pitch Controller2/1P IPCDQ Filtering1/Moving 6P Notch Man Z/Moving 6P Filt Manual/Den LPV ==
  rot speed (rad/s) : Inport
  1-D Lookup Table : Lookup_n-D  NumberOfTableDimensions=1  BreakpointsForDimension1=Parameter.Control.cIPC.PSM0_NF_6P.om_6P  BeginIndexSearchUsingPreviousIndexResult=on  Table=Parameter.Control.cIPC.PSM0_NF_6P.a_2  ExtrapMethod=Clip  InternalRulePriority=Speed  RndMeth=Simplest
  1-D Lookup Table1 : Lookup_n-D  NumberOfTableDimensions=1  BreakpointsForDimension1=Parameter.Control.cIPC.PSM0_NF_6P.om_6P  BeginIndexSearchUsingPreviousIndexResult=on  Table=Parameter.Control.cIPC.PSM0_NF_6P.a_1  ExtrapMethod=Clip  InternalRulePriority=Speed  RndMeth=Simplest
  1-D Lookup Table2 : Lookup_n-D  NumberOfTableDimensions=1  BreakpointsForDimension1=Parameter.Control.cIPC.PSM0_NF_6P.om_6P  BeginIndexSearchUsingPreviousIndexResult=on  Table=Parameter.Control.cIPC.PSM0_NF_6P.a_0  ExtrapMethod=Clip  InternalRulePriority=Speed  RndMeth=Simplest
  Mux : Mux  Inputs=3
  a : Outport
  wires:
  1-D Lookup Table/1 -> Mux/1
  1-D Lookup Table1/1 -> Mux/2
  Mux/1 -> a/1
  rot speed (rad/s)/1 -> 1-D Lookup Table2/1, 1-D Lookup Table/1, 1-D Lookup Table1/1
  1-D Lookup Table2/1 -> Mux/3

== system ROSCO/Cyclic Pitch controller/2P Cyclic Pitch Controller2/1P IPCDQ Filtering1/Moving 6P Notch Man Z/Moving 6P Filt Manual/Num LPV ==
  rot speed (rad/s) : Inport
  1-D Lookup Table : Lookup_n-D  NumberOfTableDimensions=1  BreakpointsForDimension1=Parameter.Control.cIPC.PSM0_NF_6P.om_6P  BeginIndexSearchUsingPreviousIndexResult=on  Table=Parameter.Control.cIPC.PSM0_NF_6P.b_2  ExtrapMethod=Clip  InternalRulePriority=Speed  RndMeth=Simplest
  1-D Lookup Table1 : Lookup_n-D  NumberOfTableDimensions=1  BreakpointsForDimension1=Parameter.Control.cIPC.PSM0_NF_6P.om_6P  BeginIndexSearchUsingPreviousIndexResult=on  Table=Parameter.Control.cIPC.PSM0_NF_6P.b_1  ExtrapMethod=Clip  InternalRulePriority=Speed  RndMeth=Simplest
  1-D Lookup Table2 : Lookup_n-D  NumberOfTableDimensions=1  BreakpointsForDimension1=Parameter.Control.cIPC.PSM0_NF_6P.om_6P  BeginIndexSearchUsingPreviousIndexResult=on  Table=Parameter.Control.cIPC.PSM0_NF_6P.b_0  ExtrapMethod=Clip  InternalRulePriority=Speed  RndMeth=Simplest
  Mux : Mux  Inputs=3
  b : Outport
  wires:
  1-D Lookup Table2/1 -> Mux/3
  rot speed (rad/s)/1 -> 1-D Lookup Table1/1, 1-D Lookup Table/1, 1-D Lookup Table2/1
  Mux/1 -> b/1
  1-D Lookup Table1/1 -> Mux/2
  1-D Lookup Table/1 -> Mux/1

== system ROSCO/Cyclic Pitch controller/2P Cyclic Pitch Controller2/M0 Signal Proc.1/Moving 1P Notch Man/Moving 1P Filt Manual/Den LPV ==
  rot speed (rad/s) : Inport
  1-D Lookup Table : Lookup_n-D  NumberOfTableDimensions=1  BreakpointsForDimension1=Parameter.Control.cIPC.PSM0_NF_1P.om_1P  BeginIndexSearchUsingPreviousIndexResult=on  Table=Parameter.Control.cIPC.PSM0_NF_1P.a_2  ExtrapMethod=Clip  InternalRulePriority=Speed  RndMeth=Simplest
  1-D Lookup Table1 : Lookup_n-D  NumberOfTableDimensions=1  BreakpointsForDimension1=Parameter.Control.cIPC.PSM0_NF_1P.om_1P  BeginIndexSearchUsingPreviousIndexResult=on  Table=Parameter.Control.cIPC.PSM0_NF_1P.a_1  ExtrapMethod=Clip  InternalRulePriority=Speed  RndMeth=Simplest
  1-D Lookup Table2 : Lookup_n-D  NumberOfTableDimensions=1  BreakpointsForDimension1=Parameter.Control.cIPC.PSM0_NF_1P.om_1P  BeginIndexSearchUsingPreviousIndexResult=on  Table=Parameter.Control.cIPC.PSM0_NF_1P.a_0  ExtrapMethod=Clip  InternalRulePriority=Speed  RndMeth=Simplest
  Mux : Mux  Inputs=3
  a : Outport
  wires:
  1-D Lookup Table2/1 -> Mux/3
  rot speed (rad/s)/1 -> 1-D Lookup Table1/1, 1-D Lookup Table/1, 1-D Lookup Table2/1
  Mux/1 -> a/1
  1-D Lookup Table1/1 -> Mux/2
  1-D Lookup Table/1 -> Mux/1

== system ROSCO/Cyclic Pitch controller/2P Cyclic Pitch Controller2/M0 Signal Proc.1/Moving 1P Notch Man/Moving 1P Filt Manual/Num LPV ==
  rot speed (rad/s) : Inport
  1-D Lookup Table : Lookup_n-D  NumberOfTableDimensions=1  BreakpointsForDimension1=Parameter.Control.cIPC.PSM0_NF_1P.om_1P  BeginIndexSearchUsingPreviousIndexResult=on  Table=Parameter.Control.cIPC.PSM0_NF_1P.b_2  ExtrapMethod=Clip  InternalRulePriority=Speed  RndMeth=Simplest
  1-D Lookup Table1 : Lookup_n-D  NumberOfTableDimensions=1  BreakpointsForDimension1=Parameter.Control.cIPC.PSM0_NF_1P.om_1P  BeginIndexSearchUsingPreviousIndexResult=on  Table=Parameter.Control.cIPC.PSM0_NF_1P.b_1  ExtrapMethod=Clip  InternalRulePriority=Speed  RndMeth=Simplest
  1-D Lookup Table2 : Lookup_n-D  NumberOfTableDimensions=1  BreakpointsForDimension1=Parameter.Control.cIPC.PSM0_NF_1P.om_1P  BeginIndexSearchUsingPreviousIndexResult=on  Table=Parameter.Control.cIPC.PSM0_NF_1P.b_0  ExtrapMethod=Clip  InternalRulePriority=Speed  RndMeth=Simplest
  Mux : Mux  Inputs=3
  b : Outport
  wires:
  1-D Lookup Table/1 -> Mux/1
  1-D Lookup Table1/1 -> Mux/2
  Mux/1 -> b/1
  rot speed (rad/s)/1 -> 1-D Lookup Table2/1, 1-D Lookup Table/1, 1-D Lookup Table1/1
  1-D Lookup Table2/1 -> Mux/3

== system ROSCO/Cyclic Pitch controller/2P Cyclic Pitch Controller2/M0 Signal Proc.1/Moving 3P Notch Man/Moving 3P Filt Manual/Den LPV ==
  rot speed (rad/s) : Inport
  1-D Lookup Table : Lookup_n-D  NumberOfTableDimensions=1  BreakpointsForDimension1=Parameter.Control.cIPC.PSM0_NF_3P.om_3P  BeginIndexSearchUsingPreviousIndexResult=on  Table=Parameter.Control.cIPC.PSM0_NF_3P.a_2  ExtrapMethod=Clip  InternalRulePriority=Speed  RndMeth=Simplest
  1-D Lookup Table1 : Lookup_n-D  NumberOfTableDimensions=1  BreakpointsForDimension1=Parameter.Control.cIPC.PSM0_NF_3P.om_3P  BeginIndexSearchUsingPreviousIndexResult=on  Table=Parameter.Control.cIPC.PSM0_NF_3P.a_1  ExtrapMethod=Clip  InternalRulePriority=Speed  RndMeth=Simplest
  1-D Lookup Table2 : Lookup_n-D  NumberOfTableDimensions=1  BreakpointsForDimension1=Parameter.Control.cIPC.PSM0_NF_3P.om_3P  BeginIndexSearchUsingPreviousIndexResult=on  Table=Parameter.Control.cIPC.PSM0_NF_3P.a_0  ExtrapMethod=Clip  InternalRulePriority=Speed  RndMeth=Simplest
  Mux : Mux  Inputs=3
  a : Outport
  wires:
  1-D Lookup Table/1 -> Mux/1
  1-D Lookup Table1/1 -> Mux/2
  Mux/1 -> a/1
  rot speed (rad/s)/1 -> 1-D Lookup Table2/1, 1-D Lookup Table/1, 1-D Lookup Table1/1
  1-D Lookup Table2/1 -> Mux/3

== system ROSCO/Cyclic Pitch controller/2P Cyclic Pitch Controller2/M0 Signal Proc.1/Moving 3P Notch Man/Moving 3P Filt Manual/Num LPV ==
  rot speed (rad/s) : Inport
  1-D Lookup Table : Lookup_n-D  NumberOfTableDimensions=1  BreakpointsForDimension1=Parameter.Control.cIPC.PSM0_NF_3P.om_3P  BeginIndexSearchUsingPreviousIndexResult=on  Table=Parameter.Control.cIPC.PSM0_NF_3P.b_2  ExtrapMethod=Clip  InternalRulePriority=Speed  RndMeth=Simplest
  1-D Lookup Table1 : Lookup_n-D  NumberOfTableDimensions=1  BreakpointsForDimension1=Parameter.Control.cIPC.PSM0_NF_3P.om_3P  BeginIndexSearchUsingPreviousIndexResult=on  Table=Parameter.Control.cIPC.PSM0_NF_3P.b_1  ExtrapMethod=Clip  InternalRulePriority=Speed  RndMeth=Simplest
  1-D Lookup Table2 : Lookup_n-D  NumberOfTableDimensions=1  BreakpointsForDimension1=Parameter.Control.cIPC.PSM0_NF_3P.om_3P  BeginIndexSearchUsingPreviousIndexResult=on  Table=Parameter.Control.cIPC.PSM0_NF_3P.b_0  ExtrapMethod=Clip  InternalRulePriority=Speed  RndMeth=Simplest
  Mux : Mux  Inputs=3
  b : Outport
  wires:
  1-D Lookup Table2/1 -> Mux/3
  rot speed (rad/s)/1 -> 1-D Lookup Table1/1, 1-D Lookup Table/1, 1-D Lookup Table2/1
  Mux/1 -> b/1
  1-D Lookup Table1/1 -> Mux/2
  1-D Lookup Table/1 -> Mux/1

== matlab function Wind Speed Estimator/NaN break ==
function y = fcn(u)

if isnan(u)
    a = 1;
end

y = u;

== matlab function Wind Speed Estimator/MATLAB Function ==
function [vh,xh,P,K,Debug] = WSE_EKF(omega_r, tau_g, beta, WE_params, A_op, xh,P,K,dt,t,HorWind, Cx)
% This function defines a WSE based off of an Extended Kalman Filter
% Inputs:
% Outputs:
% Nikhar Abbas

% Load R variables
J       = WE_params(1);                    % Rotor Inertia
rho     = WE_params(2);                % Air density
Rr      = WE_params(3);             % Rotor Radius, R
Ng      = WE_params(4);             % Gearbox Ratio

% Simulink Offset, between mean wind speeds due to poor startup transients
sOff    = 0.8;

% Constants
H       = [1 0 0];
R       = 0.02;
L       = 6 * Rr;
Ti      = 0.2;
A       = pi*Rr^2;                         % Rotor Swept Area, m^2


% organize Inputs
if t < dt
    om_r    = omega_r;
    v_t     = 0;
    v_m     = HorWind + sOff;
else
    om_r    = xh(1);
    v_t     = xh(2);
    v_m     = xh(3) + sOff;
end

om_m    = omega_r;

% Debug Outs
Debug   = zeros(2,1);

% Find current estimated operating conditions, and saturate
v_r     = v_t + v_m;
lambda  = om_m * Rr / v_r;
lambda  = max( min(lambda, Cx.TSR(end)), Cx.TSR(1));


% A_op (system pole) interpolation
% A_op    = interp1(R.WE_FOPoles_v,R.WE_FOPoles,xh(1) + xh(2));


% Cp interpolation
Cp      = interp2(Cx.BlPitch,Cx.TSR,Cx.Cpmat,beta * rad2deg(1),lambda);
Cp      = max(0,Cp);


% Calculate Jacobians
F       = zeros(3,3);

F(1,1)      = A_op;
F(1,2)      = 1/(2*J)*rho*A*Cp*3*(v_m+v_t)^2*1/om_r;
F(1,3)      = 1/(2*J)*rho*A*Cp*3*(v_m+v_t)^2*1/om_r;

F(2,2)      = pi * v_m / (2*L);
F(2,3)      = pi * v_t / (2*L);  % this was 0


% Calculate Covariance
Q           = zeros(3,3);
Q(1,1)      = 1e-5;                     %in DZ WSE, 1e-6
Q(2,2)      = pi * v_m^3 * Ti^2 / L;
Q(3,3)      = 2^2/600;


%% Prediction Update

% states
tau_r       = 1/2 * rho * A * Cp * v_r^3 / om_m;       % Torque calculation
tau_r       = max(tau_r,0);
a           = pi * v_m / (2 * L);                           % Wind variance
dom_r       = 1/J * (tau_r - Ng * tau_g);
dv_t        = -a*v_t;
dv_m        = 0;
dxh         = [dom_r; dv_t; dv_m];

% forward euler
xh          = xh + dt*dxh;

% covariance
dP          = F*P + P*F' + Q - K*R*K';
P           = P + dt*dP;

% kalman gain
S           = H*P*H' + R;
K           = P * H' / S(1,1);   %DZ: this is odd, keep an eye on
% K           = P * H' * inv(S);   %DZ: this is odd, keep an eye on...was probably giving NJA stability issues

% output residual & update
y_til       = om_m - om_r;
xh          = xh + K*y_til;
P           = (eye(3) - K * H) * P;         % DZ: this is also different, but I think I've seen this form before


% Output Wind Speed Estimate
vh = v_m + v_t;

% Set Debug Outputs
Debug(1) = Cp;
Debug(2) = v_m;
end

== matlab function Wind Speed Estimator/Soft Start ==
function out = softStart(startTime,endTime,time,generic,actual)

as  = Af_sigma(startTime,endTime);
T   = [time^3,time^2,time,1]';

if time < startTime
    act = 0;
    gen = 1;
elseif time >= startTime && time < endTime
    act = as * T; 
    gen = 1 - as * T;
else
    act = 1;
    gen = 0;
end

out = act*actual + gen*generic;

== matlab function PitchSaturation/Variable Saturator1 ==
function [pitchCommandOut,atLimit] = variableSat(pitchCommand,lowerLimit,upperLimit)
%#codegen

if pitchCommand < lowerLimit
    pitchCommandOut = lowerLimit;
    atLimit          = 1;
    
elseif pitchCommand > upperLimit
    pitchCommandOut = upperLimit;
    atLimit         = 1;
    
else
    pitchCommandOut = pitchCommand;
    atLimit         = 0;
end

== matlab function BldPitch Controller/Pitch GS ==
function [Ki, Kp] = GainSchedule(Beta, Kp_pc, Ki_pc,  PC_beta)

% This function calculates the current gains for a Collective Blade Pitch 
% controller
%
% Inputs: v - Current wind speed estimate, m/s.
%         ContParam - Structure of control parameters, output from
%                     ControlParameters.m
%
% Outputs: Kp - Proportional Gain
%          Ki - Integral Gain
%
% Nikhar Abbas - May 2019


%% Linear Gain Schedule
% pKp_pc = ContParam.GS.pKp_pc;
% pKi_pc = ContParam.GS.pKi_pc;
% 
% %%
% Kp = pKp_pc(1)*Beta + pKp_pc(2);
% Ki = pKi_pc(1)*Beta + pKi_pc(2);
% % Kp = pKp_pc(1)*v + pKp_pc(2)
% % Ki = pKi_pc(1)*v + pKi_pc(2);
% 
% Kpmax = pKp_pc(1)*15*pi/180 + pKp_pc(2);
% Kimax = pKi_pc(1)*15*pi/180 + pKi_pc(2);
% 
% Kp = min(Kp, Kpmax);
% Ki = min(Ki,Kimax);

%% nonlinear Gain Schedule
% Kp_pc   = R.PC_GS_KP;
% Ki_pc   = R.PC_GS_KI;
% PC_beta = R.PC_GS_angles;

beta    = max(min(Beta,PC_beta(end)), PC_beta(1));

% gains
Kp      = interp1(PC_beta,Kp_pc, beta);
Ki      = interp1(PC_beta,Ki_pc, beta);



end

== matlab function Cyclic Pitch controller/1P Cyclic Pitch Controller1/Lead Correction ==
function [b_cos,b_sin] = fcn(bdq, psi_o)
% This block supports the Embedded MATLAB subset.
% See the help menu for details. 

b_cos=[cosd(psi_o) sind(psi_o)]*bdq;
b_sin=[-sind(psi_o) cosd(psi_o)]*bdq;

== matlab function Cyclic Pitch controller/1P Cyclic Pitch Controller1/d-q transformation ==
function [M_tilt,M_yaw] = fwdMBC2(RootMyb, Az, NumBl)
% This block supports the Embedded MATLAB subset.
% See the help menu for details.

if NumBl == 2
    
    My=RootMyb-mean(RootMyb(1:2)); %remove mean
    
    M_tilt = [cosd(Az) cosd(Az+180) 0]*My;
    M_yaw =  [sind(Az) sind(Az+180) 0]*My;
else
    My=RootMyb-mean(RootMyb); %remove mean
    
    M_tilt = [cosd(Az) cosd(Az+120) cosd(Az+240)]*My;
    M_yaw =  [sind(Az) sind(Az+120) sind(Az+240)]*My;
end

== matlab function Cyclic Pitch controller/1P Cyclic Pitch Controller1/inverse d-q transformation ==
function [b1,b2,b3] = bckMBC2(bdq, Az, NumBl)
% This block supports the Embedded MATLAB subset.
% See the help menu for details.


if NumBl == 2
    
    b1=[cosd(Az) sind(Az)]*bdq;
    b2=[cosd(Az - 180) sind(Az - 180)]*bdq;
    b3=0;
    
else
    b1=[cosd(Az) sind(Az)]*bdq;
    b2=[cosd(Az + 120) sind(Az + 120)]*bdq;
    b3=[cosd(Az + 240) sind(Az + 240)]*bdq;
    
end
